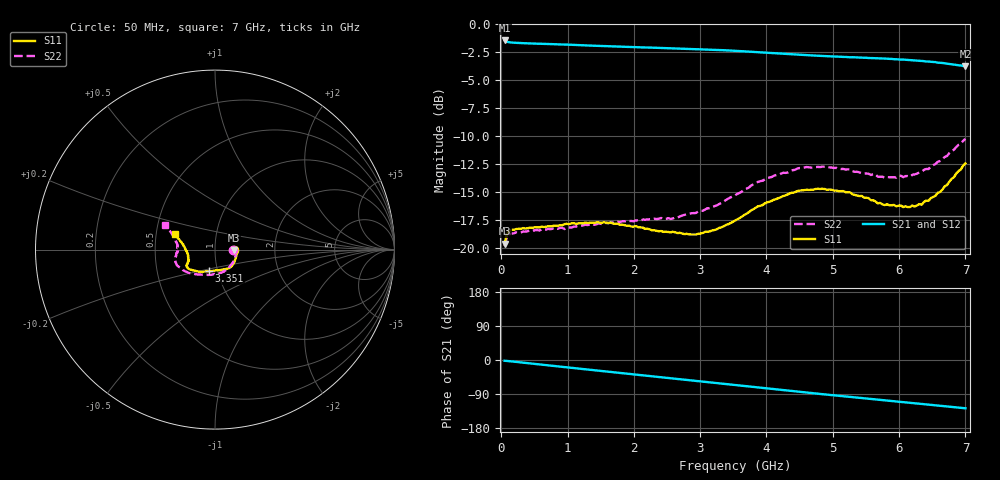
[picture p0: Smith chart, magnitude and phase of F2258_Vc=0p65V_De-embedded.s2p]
! Integrated Device Technology
! Corporate Headquarters
! 6024 Silver Creek Valley Road
! San Jose, CA 95138  USA
! Phone:  1-408-284-8200
! Toll Free:  1-800-223-1366
! Webpage:  http://www.idt.com/
! Timing and RF Division
! 515 Groton Road, Suite 102
! Westford, MA 01886-6024
! Device:  F2258
! Description: Voltage Variable RF Attenuator
! Frequency:  50.0 -  6000.00 MHz
! Package:  3x3 mm Thin QFN Plastic Package: 16 pin
! Ports:  2 RF, 2 DC
!  Pin  1  = NC
!  Pin  2  = NC
!  Pin  3  = RF2  = Port 2
!  Pin  4  = GND
!  Pin  5  = Vdd
!  Pin  6  = NC
!  Pin  7  = VCTRL
!  Pin  8  = NC
!  Pin  9  = GND
!  Pin 10  = RF1  = Port 1
!  Pin 11  = NC
!  Pin 12  = NC
!  Pin 13  = NC
!  Pin 14  = NC
!  Pin 15  = NC
!  Pin 16  = NC
! Vcntrl:  0.650 Volts
! Vdd:  +3.300 Volts
! Current:  1.113 mA
! Data:  The device was measured on a the F2258 evaluation board which has
!  individual transmission lines to the RF pins.  Data was collected
!  using a calibrated network analyzer.  The evaluation board was
!  de-embedded using a TRL calibration technique.
!  The reference plane is the edge of the package pin.
! Misc:  SN 10
!  Action Tracker AT0285
! Date Measured:  2014-12-10
! Date:  2016-01-13  MJV
! Note:
!  Integrated Device Technology supplies this data as a sample of measured
!  data at the package pin for this product.  Your particular data for this
!  product may vary.
!  Data was taken at 25 degrees C.
!  Integrated Device Technology reserves the right to change this data at anytime.
!Freq_(GHz)  S11M_(dB)  S11P_(deg)  S21M_(dB)  S21P_(deg)  S12M_(dB)  S12P_(deg)  S22M_(dB)  S22P_(deg)
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# GHz S dB R 50
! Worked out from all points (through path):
!   201 points, 50 MHz to 7 GHz, reference 50 ohm
!   highest |S21| = -1.45 dB at 50 MHz (marker M1); lowest = -3.8 dB at 7 GHz (marker M2)
!   group delay of S21, straight-line fit = 50.5 ps
!   lowest |S11| = -19.6 dB at 50 MHz (marker M3), VSWR 1.24, Z = 61.7 - j0.494 ohm
!   |S11| at or under -10 dB: start of sweep to end of sweep
!   |S22| runs from -19.8 to -10.2 dB; largest |S21 - S12| = 0.0013
!   S11 on the Smith chart (normalised r, x): 50 MHz: 1.23, -0.01; 3.351 GHz: 0.91, -0.22; 7 GHz: 0.63, +0.11
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0.05  -19.56 -2.2  -1.45 -2.0  -1.45 -2.0  -19.79 -2.7
0.08475  -18.73 -3.6  -1.56 -2.5  -1.56 -2.5  -18.96 -4.2
0.15425  -18.34 -5.8  -1.63 -3.7  -1.63 -3.7  -18.66 -7.4
0.71025  -18.01 -25.1  -1.77 -14.2  -1.77 -14.2  -18.25 -30.8
0.9535  -17.83 -34.1  -1.81 -18.8  -1.82 -18.8  -18.27 -42.1
1.2315  -17.76 -41.8  -1.88 -23.9  -1.89 -23.9  -17.95 -52.3
1.6485  -17.68 -51.3  -1.98 -31.5  -1.98 -31.5  -17.68 -65.3
2.37825  -18.46 -67.2  -2.11 -44.8  -2.12 -44.8  -17.35 -84.7
2.58675  -18.51 -73.1  -2.15 -48.6  -2.16 -48.6  -17.33 -91.3
2.93425  -18.76 -86.6  -2.22 -55.1  -2.23 -55.1  -16.84 -103.7
3.35125  -18.04 -105.6  -2.32 -63.0  -2.33 -63.0  -15.84 -120.4
3.525  -17.52 -113.6  -2.37 -66.3  -2.38 -66.3  -15.27 -127.3
4.0115  -15.88 -132.1  -2.55 -75.3  -2.56 -75.3  -13.72 -144.1
4.46325  -14.89 -142.7  -2.72 -83.5  -2.72 -83.5  -12.88 -156.0
4.7065  -14.75 -146.2  -2.79 -87.8  -2.80 -87.8  -12.78 -160.7
5.2625  -15.00 -152.3  -2.95 -97.4  -2.95 -97.4  -12.95 -169.6
5.6795  -15.98 -157.0  -3.04 -104.6  -3.04 -104.5  -13.60 -175.7
5.85325  -16.15 -160.9  -3.09 -107.7  -3.09 -107.7  -13.65 179.5
6.166  -16.30 -169.2  -3.19 -113.2  -3.20 -113.2  -13.59 173.0
6.33975  -16.10 -176.7  -3.28 -116.3  -3.28 -116.3  -13.16 168.4
6.61775  -14.96 170.9  -3.44 -121.2  -3.44 -121.2  -12.20 161.5
7  -12.42 159.0  -3.76 -127.4  -3.76 -127.4  -10.21 153.5
